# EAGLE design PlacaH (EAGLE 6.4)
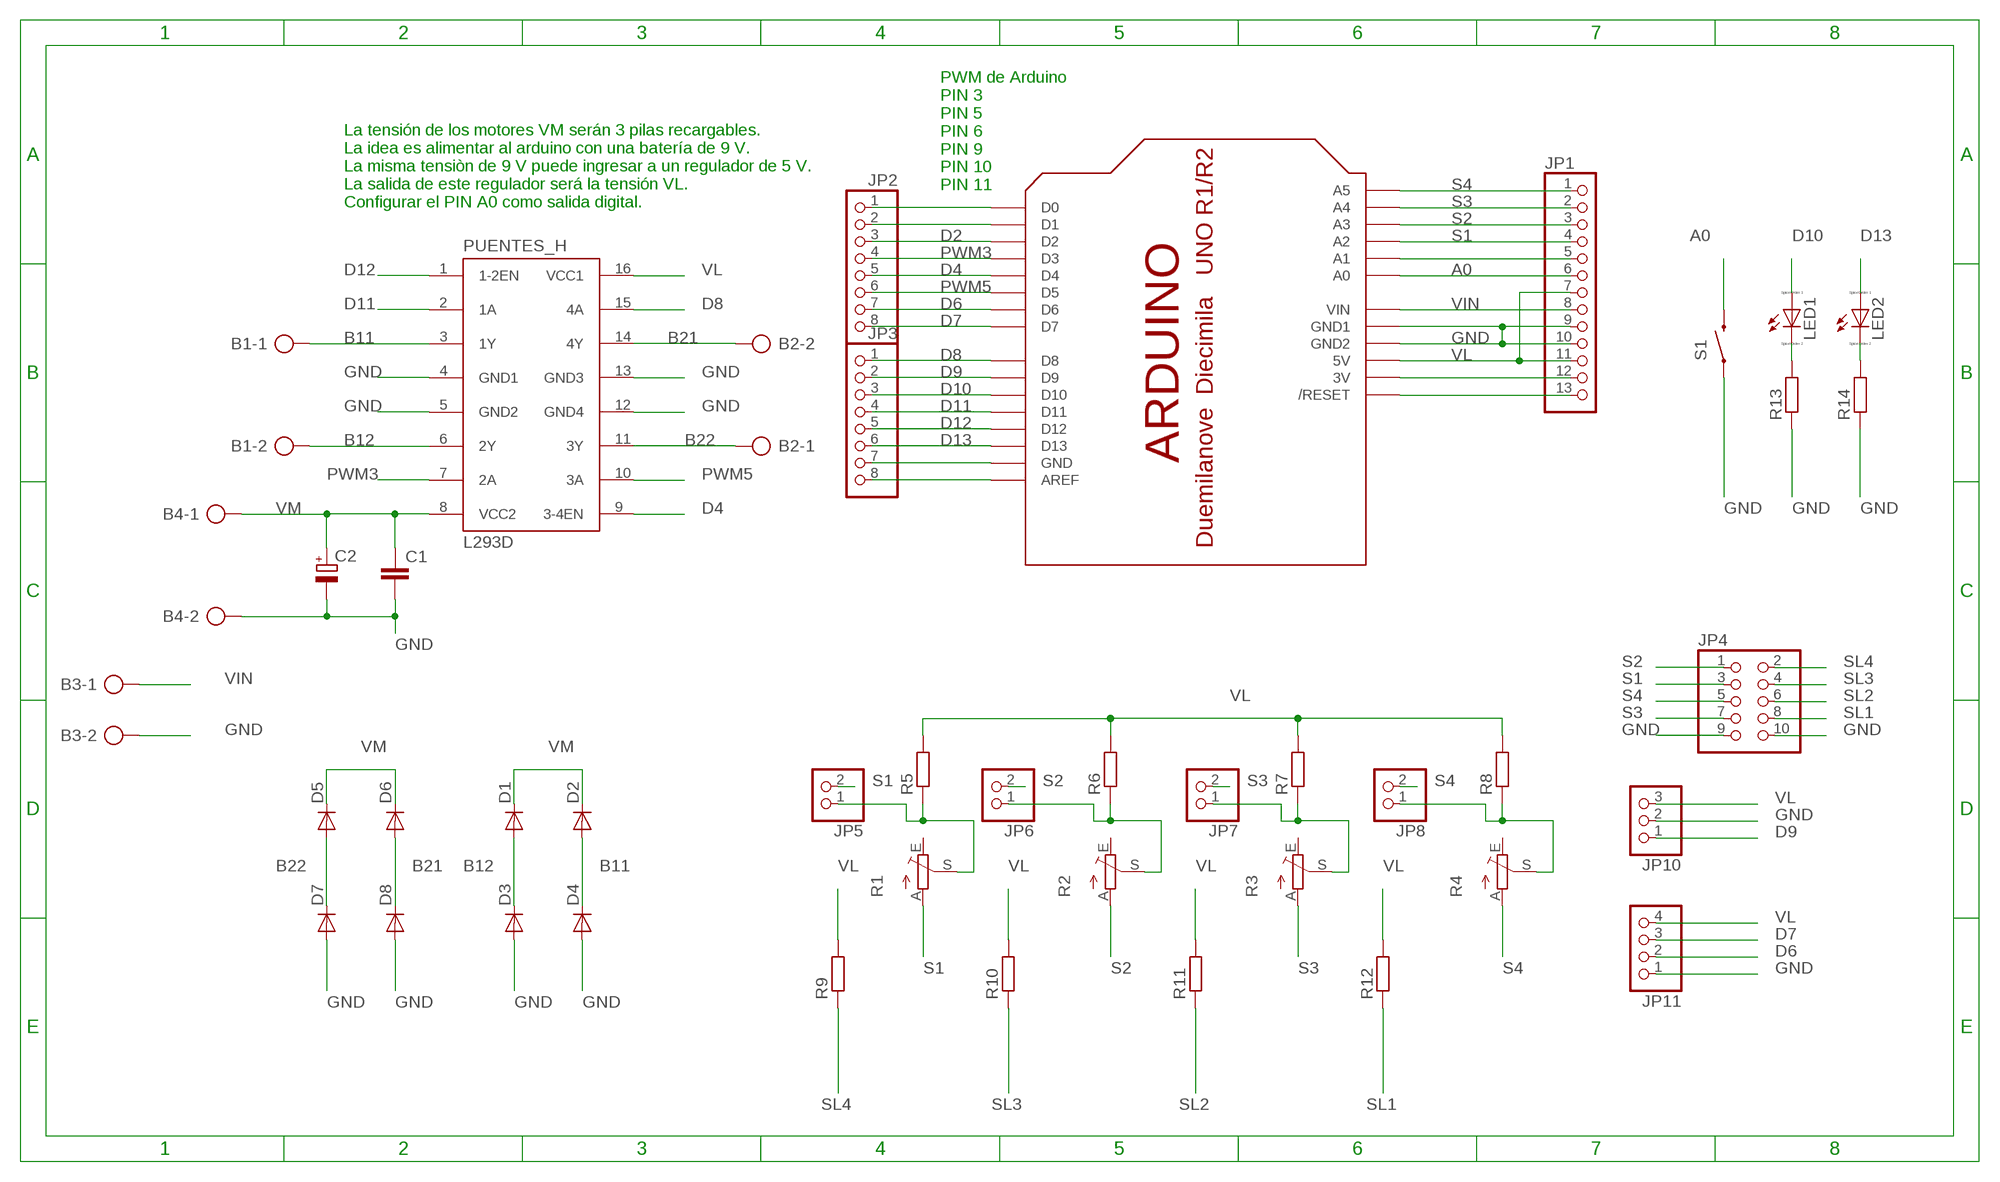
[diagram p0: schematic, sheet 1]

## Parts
B1  AK500/2-H  [AK500/2-H]
B2  AK500/2-H  [AK500/2-H]
B3  AK500/2-H  [AK500/2-H]
B4  AK500/2-H  [AK500/2-H]
C1  C-EUC1808  [C1808]
C2  CPOL-EUE2.5-6  [E2,5-6]
D1  CGRM4007-G  [SOD-123_MINI-SMA]
D2  CGRM4007-G  [SOD-123_MINI-SMA]
D3  CGRM4007-G  [SOD-123_MINI-SMA]
D4  CGRM4007-G  [SOD-123_MINI-SMA]
D5  CGRM4007-G  [SOD-123_MINI-SMA]
D6  CGRM4007-G  [SOD-123_MINI-SMA]
D7  CGRM4007-G  [SOD-123_MINI-SMA]
D8  CGRM4007-G  [SOD-123_MINI-SMA]
JP1  PINHD-1X13  [1X13]
JP2  PINHD-1X8  [1X08]
JP3  PINHD-1X8  [1X08]
JP4  PINHD-2X5  [2X05]
JP5  PINHD-1X2  [1X02]
JP6  PINHD-1X2  [1X02]
JP7  PINHD-1X2  [1X02]
JP8  PINHD-1X2  [1X02]
JP10  PINHD-1X3  [1X03]
JP11  PINHD-1X4  [1X04]
LED1  LED_E  [LED_1206]
LED2  LED_E  [LED_1206]
PUENTES_H  L293D  [DIL16]
R1  TRIM_EU-B25P  [B25P]
R2  TRIM_EU-B25P  [B25P]
R3  TRIM_EU-B25P  [B25P]
R4  TRIM_EU-B25P  [B25P]
R5  R-EU_M1206  [M1206]
R6  R-EU_M1206  [M1206]
R7  R-EU_M1206  [M1206]
R8  R-EU_M1206  [M1206]
R9  R-EU_M1206  [M1206]
R10  R-EU_M1206  [M1206]
R11  R-EU_M1206  [M1206]
R12  R-EU_M1206  [M1206]
R13  R-EU_M1206  [M1206]
R14  R-EU_M1206  [M1206]
S1  SWITCH-MOMENTARY-2PTH  [TACTILE-PTH]
U$1  ARDUINO-BPLACE  [ARDUINO-BPLACE]

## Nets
A0: JP1.6 S1.3 U$1.A0
B11: B1.1 D2.A D4.C PUENTES_H.3(1Y)
B12: B1.2 D1.A D3.C PUENTES_H.6(2Y)
B21: B2.2 D6.A D8.C PUENTES_H.14(4Y)
B22: B2.1 D5.A D7.C PUENTES_H.11(3Y)
D2: JP2.3 U$1.D2
D4: JP2.5 PUENTES_H.9(3-4EN) U$1.D4
D6: JP2.7 JP11.2 U$1.D6
D7: JP2.8 JP11.3 U$1.D7
D8: JP3.1 PUENTES_H.15(4A) U$1.D8
D9: JP3.2 JP10.1 U$1.D9
D10: JP3.3 LED1.A U$1.D10
D11: JP3.4 PUENTES_H.2(1A) U$1.D11
D12: JP3.5 PUENTES_H.1(1-2EN) U$1.D12
D13: JP3.6 LED2.A U$1.D13
GND: B3.2 B4.2 C1.2 C2.- D3.A D4.A D7.A D8.A JP1.9 JP1.10 JP4.9 JP4.10 JP10.2 JP11.1 PUENTES_H.4(GND1) PUENTES_H.5(GND2) PUENTES_H.12(GND4) PUENTES_H.13(GND3) R13.1 R14.1 S1.1 U$1.GND1 U$1.GND2
N$5: JP5.1 R1.S R5.1
N$7: JP6.1 R2.S R6.1
N$8: JP7.1 R3.S R7.1
N$9: JP8.1 R4.S R8.1
N$48: JP1.13 U$1.RESET(/RESET)
N$49: JP1.12 U$1.3V
N$51: JP1.5 U$1.A1
N$72: JP2.1 U$1.D0
N$73: JP2.2 U$1.D1
N$75: LED1.C R13.2
N$76: JP3.7 U$1.GND
N$77: JP3.8 U$1.AREF
N$163: LED2.C R14.2
PWM3: JP2.4 PUENTES_H.7(2A) U$1.D3
PWM5: JP2.6 PUENTES_H.10(3A) U$1.D5
S1: JP1.4 JP4.3 JP5.2 R1.A U$1.A2
S2: JP1.3 JP4.1 JP6.2 R2.A U$1.A3
S3: JP1.2 JP4.7 JP7.2 R3.A U$1.A4
S4: JP1.1 JP4.5 JP8.2 R4.A U$1.A5
SL1: JP4.8 R12.1
SL2: JP4.6 R11.1
SL3: JP4.4 R10.1
SL4: JP4.2 R9.1
VIN: B3.1 JP1.8 U$1.VIN
VL: JP1.7 JP1.11 JP10.3 JP11.4 PUENTES_H.16(VCC1) R5.2 R6.2 R7.2 R8.2 R9.2 R10.2 R11.2 R12.2 U$1.5V
VM: B4.1 C1.1 C2.+ D1.C D2.C D5.C D6.C PUENTES_H.8(VCC2)
Unconnected: R1.E R2.E R3.E R4.E

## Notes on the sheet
- PWM de Arduino
  PIN 3
  PIN 5
  PIN 6
  PIN 9
  PIN 10
  PIN 11
- La tensión de los motores VM serán 3 pilas recargables.
  La idea es alimentar al arduino con una batería de 9 V.
  La misma tensiòn de 9 V puede ingresar a un regulador de 5 V.
  La salida de este regulador será la tensión VL.
  Configurar el PIN A0 como salida digital.

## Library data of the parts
B1-B4 = con-ptr500:AK500/2-H: CONNECTOR; OC_FARNELL: unknown; OC_NEWARK: unknown
C1 = rcl:C-EU: CAPACITOR, European symbol
C2 = rcl:CPOL-EU: POLARIZED CAPACITOR, European symbol
D1-D8 = diode:CGRM400*-G: Molded plasitc,JEDEC SOD-123/Mini SMA
JP1 = pinhead:PINHD-1X13: PIN HEADER
JP2 JP3 = pinhead:PINHD-1X8: PIN HEADER
JP4 = pinhead:PINHD-2X5: PIN HEADER
JP5-JP8 = pinhead:PINHD-1X2: PIN HEADER
JP10 = pinhead:PINHD-1X3: PIN HEADER
JP11 = pinhead:PINHD-1X4: PIN HEADER
LED1 LED2 = eagle-ltspice:LED_E: LED; SPICEMODEL: NONE; SPICEPREFIX: D; SPICETYPE: diode
PUENTES_H = st-microelectronics:L293D: PUSH-PULL 4 CHANNEL DRIVER; MPN: L293D; OC_FARNELL: 9589619; OC_NEWARK: 56P8249
R1-R4 = pot:TRIM_EU-: POTENTIOMETER
R5-R14 = rcl:R-EU_: RESISTOR, European symbol
S1 = SparkFun-Electromechanical:SWITCH-MOMENTARY-2: Various NO switches- pushbuttons, reed, etc
U$1 = adafruit:ARDUINO: Arduino Diecimila/Duemilanove Make a shield with ease, this package has all the named pins as well as the two mounting drill holes and an outline of the USB and DC power connector. The outline is on the DIMENSION layer, so if your board house uses it they will cut the outline to match.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

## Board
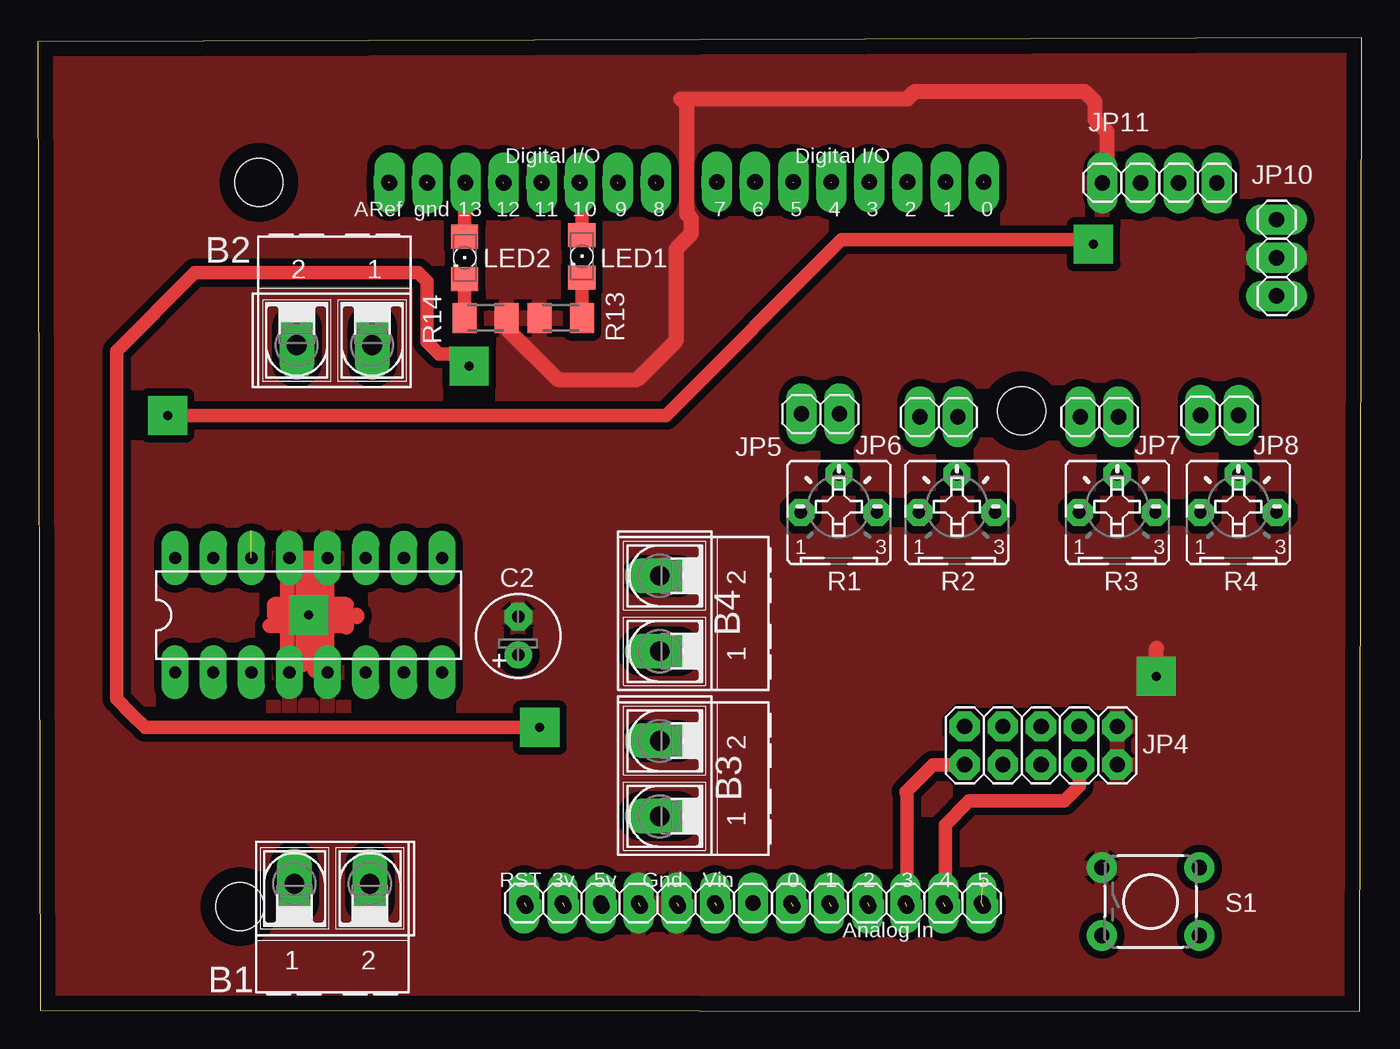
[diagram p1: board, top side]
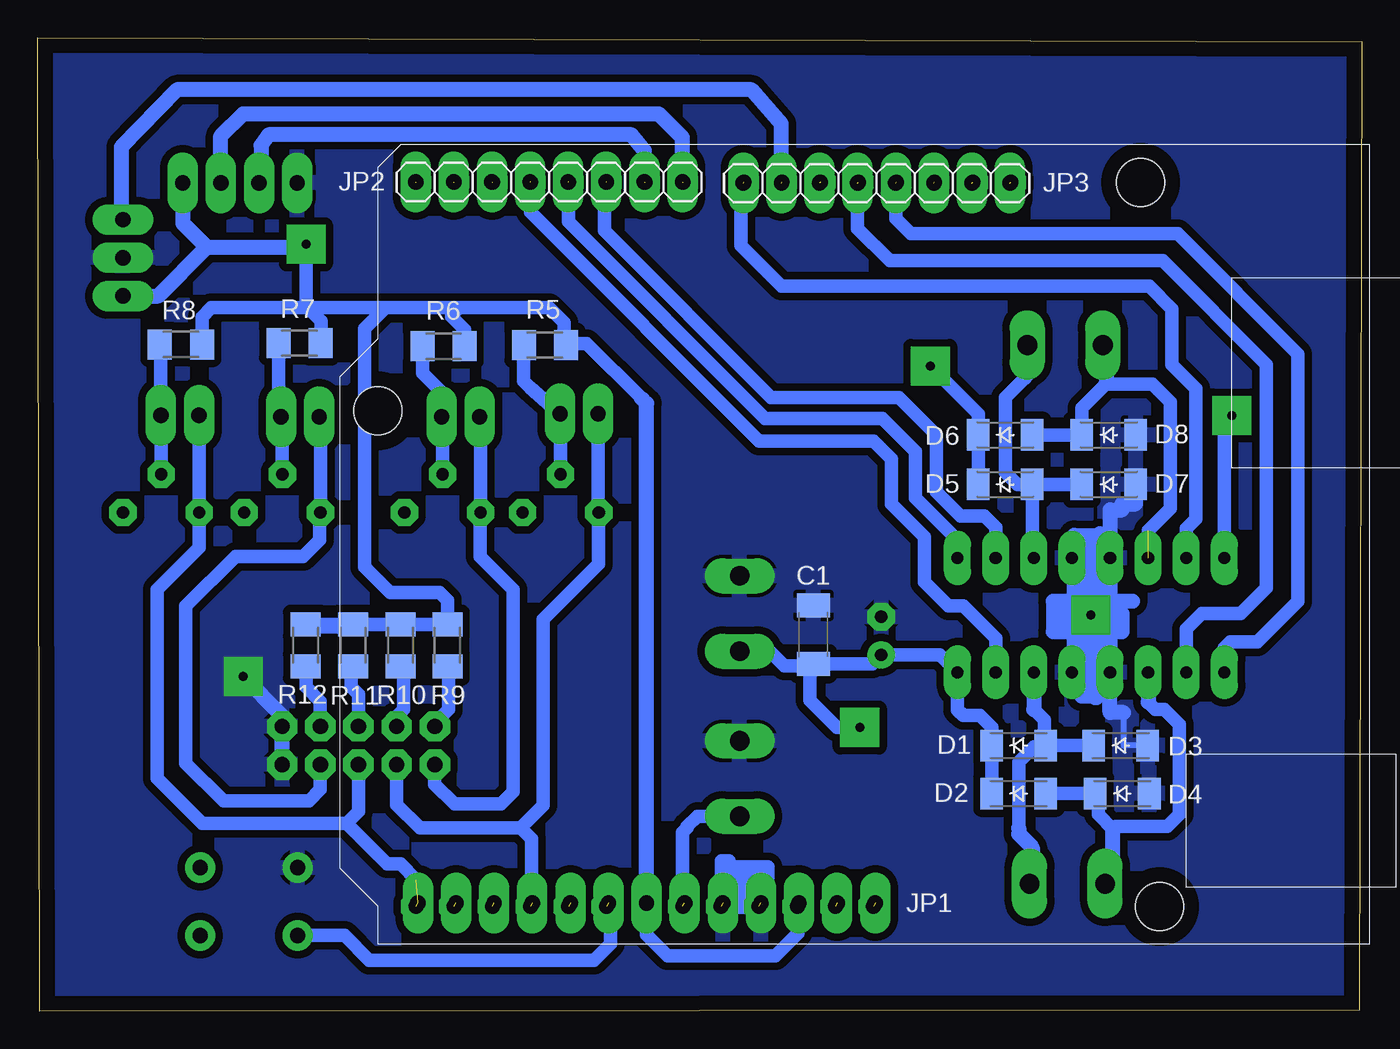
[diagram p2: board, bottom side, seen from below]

Size 88.26 x 64.91 mm. Coordinates in mm from the lower left corner, seen from the top.
Outline: 0.19,0.09 88.1,0 88.26,64.91 0,64.61 0.19,0.09
Copper layers (1*16): Top 0.035mm / dielectric 1.5mm / Bottom 0.035mm
Design rules "default *": minimum track width 1mm, minimum drill 0.01mm, track to track 0.5mm, track to pad 0.8mm, pad to pad 0.75mm, via to via 0.75mm, smd to smd 1mm, copper to edge 40mil, drill to drill 10mil, minimum pad ring 0.5mm, minimum via ring 1mm, stop-mask expansion 4mil, vias tented up to drill 0mil, thermal gap 10mil

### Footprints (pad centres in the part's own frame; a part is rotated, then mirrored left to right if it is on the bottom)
AK500/2-H = drill 1.321 long: 1 -2.515,0; 2 2.515,0
C1808 = smd 1.6 x 2.2: 1 -1.95,0; 2 1.95,0
E2,5-6 = drill 0.813 pad 1.6: + -1.27,0 | drill 0.813 pad 1.6 octagon: - 1.27,0
SOD-123_MINI-SMA = smd 1.5 x 2.1: A 1.8,0; C -1.8,0
1X13 = drill 1.016 long: 1 -15.24,0; 2 -12.7,0; 3 -10.16,0; 4 -7.62,0; 5 -5.08,0; 6 -2.54,0; 7 0,0; 8 2.54,0; 9 5.08,0; 10 7.62,0; 11 10.16,0; 12 12.7,0; 13 15.24,0
1X08 = drill 1.016 long: 1 -8.89,0; 2 -6.35,0; 3 -3.81,0; 4 -1.27,0; 5 1.27,0; 6 3.81,0; 7 6.35,0; 8 8.89,0
2X05 = drill 1.016 octagon: 1 -5.08,-1.27; 2 -5.08,1.27; 3 -2.54,-1.27; 4 -2.54,1.27; 5 0,-1.27; 6 0,1.27; 7 2.54,-1.27; 8 2.54,1.27; 9 5.08,-1.27; 10 5.08,1.27
1X02 = drill 1.016 long: 1 -1.27,0; 2 1.27,0
1X03 = drill 1.016 long: 1 -2.54,0; 2 0,0; 3 2.54,0
1X04 = drill 1.016 long: 1 -3.81,0; 2 -1.27,0; 3 1.27,0; 4 3.81,0
LED_1206 = smd 1.6 x 1.803: A -1.422,0; C 1.422,0
DIL16 = drill 0.813 long: 1 -8.89,-3.81; 2 -6.35,-3.81; 3 -3.81,-3.81; 4 -1.27,-3.81; 5 1.27,-3.81; 6 3.81,-3.81; 7 6.35,-3.81; 8 8.89,-3.81; 9 8.89,3.81; 10 6.35,3.81; 11 3.81,3.81; 12 1.27,3.81; 13 -1.27,3.81; 14 -3.81,3.81; 15 -6.35,3.81; 16 -8.89,3.81
B25P = drill 0.813 octagon: A -2.54,0; E 2.54,0; S 0,2.54
M1206 = smd 1.6 x 2: 1 -1.4,0; 2 1.4,0
TACTILE-PTH = drill 1.016 pad 1.88: 1 -3.251,2.261; 2 3.251,2.261; 3 -3.251,-2.261; 4 3.251,-2.261
ARDUINO-BPLACE = drill 1 pad 1.676 octagon: 3V 35.56,2.54; 5V 38.1,2.54; A0 50.8,2.54; A1 53.34,2.54; A2 55.88,2.54; A3 58.42,2.54; A4 60.96,2.54; A5 63.5,2.54; AREF 23.876,50.8; D0 63.5,50.8; D1 60.96,50.8; D2 58.42,50.8; D3 55.88,50.8; D4 53.34,50.8; D5 50.8,50.8; D6 48.26,50.8; D7 45.72,50.8; D8 41.656,50.8; D9 39.116,50.8; D10 36.576,50.8; D11 34.036,50.8; D12 31.496,50.8; D13 28.956,50.8; GND 26.416,50.8; GND1 43.18,2.54; GND2 40.64,2.54; RESET 33.02,2.54; VIN 45.72,2.54 | hole 3.2: 15.24,50.8; 66.04,35.56; 13.97,2.54

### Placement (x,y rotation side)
B1  19.63,8.51 0 top
B2  19.79,44.41 180 top
B3  41.47,15.52 90 top
B4  41.47,26.52 90 top
C1  36.56,25.11 90 bottom
C2  32.03,25.04 90 top
D1  22.87,17.72 0 bottom
D2  22.87,14.52 0 bottom
D3  16.07,17.72 0 bottom
D4  15.97,14.52 0 bottom
D5  23.77,35.12 0 bottom
D6  23.77,38.42 0 bottom
D7  16.87,35.12 0 bottom
D8  16.87,38.42 0 bottom
JP1  47.67,7.22 180 top
JP2  54.17,55.28 0 bottom
JP3  32.34,55.21 0 bottom
JP4  66.87,17.72 0 top
JP5  52.17,39.82 180 top
JP6  60.07,39.62 180 top
JP7  70.77,39.62 180 top
JP8  78.77,39.72 180 top
JP10  82.57,50.22 270 top
JP11  74.77,55.22 0 top
LED1  36.27,50.32 270 top
LED2  28.47,50.22 270 top
PUENTES_H  18.06,26.41 0 top
R1  53.4,33.26 0 top
R2  61.27,33.26 0 top
R3  71.95,33.26 0 top
R4  80.02,33.26 0 top
R5  54.45,44.4 0 bottom
R6  61.2,44.33 0 bottom
R7  70.8,44.55 0 bottom
R8  78.7,44.46 0 bottom
R9  60.95,24.41 90 bottom
R10  64.06,24.41 90 bottom
R11  67.23,24.41 90 bottom
R12  70.39,24.41 90 bottom
R13  34.87,46.22 0 top
R14  29.87,46.22 180 top
S1  74.17,7.32 0 top
U$1  -0.47,4.46 0 top

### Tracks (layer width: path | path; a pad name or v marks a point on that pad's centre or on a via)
A0  (1 unrouted)
  Bottom 0.9: S1.3 67.81,5.06 66.17,3.42 51.17,3.42 50.07,4.52 50.07,5.42 | 50.07,5.42 50.07,6.75 | JP1.6 50.21,5.56 50.07,5.42
B11
  Bottom 0.9: D2.A D4.C 17.57,14.32 17.57,13.12 16.59,12.14 16.41,12.32 12.97,12.32 12.17,13.12 12.17,19.12 13.17,20.12 13.77,20.12 14.25,20.6
  Bottom 1: PUENTES_H.3 14.25,20.6 | B1.1 16.59,8.51 16.59,12.14
B12
  Bottom 0.9: 21.87,20.12 21.17,19.42 21.17,17.82 D1.A | D1.A D3.C | 22.87,12.22 22.87,16.62 21.87,17.62 21.17,17.62 D1.A
  Bottom 1: PUENTES_H.6 21.87,20.12 | 21.62,8.51 B1.2 21.97,8.69 21.97,10.92 22.87,11.82 22.87,12.22
B21  (1 unrouted)
  Bottom 0.9: D6.A D8.C 18.67,40.22 17.04,41.86 17,41.82 13.97,41.82 12.77,40.62 12.77,33.52 14.25,32.04
  Bottom 1: B2.2 17.04,44.41 17.04,41.86
B22
  Bottom 0.9: D5.A 21.97,30.32 PUENTES_H.11 | D5.A D7.C | 22.07,42.63 22.47,42.22 23.77,40.92 23.77,35.92 22.97,35.12 D5.A
  Bottom 1: B2.1 22.47,44.41 22.47,42.22
D2  (1 unrouted)
D4  (1 unrouted)
  Bottom 0.9: PUENTES_H.9 26.95,31.4 29.77,34.22 29.77,37.32 31.97,39.52 39.77,39.52 52.87,52.62 U$1.D4
D6  (1 unrouted)
  Bottom 1: JP2.7 47.82,57.38 48.67,58.42 72.87,58.42 73.37,57.72 73.37,54.92 73.57,54.72 73.57,55.15 JP11.2
D7  (1 unrouted)
  Bottom 1: JP2.8 45.28,58.24 46.87,59.82 74.57,59.82 76.04,58.35 JP11.3
D8  (1 unrouted)
  Bottom 0.9: PUENTES_H.15 11.71,32.18 11.07,32.82 11.07,41.52 12.67,43.12 12.67,46.82 14.17,48.32 38.67,48.32 41.37,51.02 41.37,55.07 JP3.1
D9  (1 unrouted)
  Bottom 1: JP3.2 38.69,59.14 40.67,61.42 78.97,61.42 82.67,57.62 82.67,52.86 JP10.1
D10  (1 unrouted)
  Top 0.9: LED1.A 36.27,55.1 U$1.D10
D11  (1 unrouted)
  Bottom 0.9: PUENTES_H.2 11.71,25.48 10.67,26.52 8.07,26.52 6.37,28.22 6.37,43.12 13.27,50.02 31.47,50.02 33.61,52.16 JP3.4 33.57,55.17
D12  (1 unrouted)
  Bottom 0.9: PUENTES_H.1 9.17,24.22 8.77,24.62 6.97,24.62 4.27,27.32 4.27,43.82 12.27,51.82 30.07,51.82 31.07,52.82 JP3.5 | JP3.5
D13  (1 unrouted)
  Top 0.9: JP3.6 28.47,55.15 LED2.A
GND  (via drill 0.6)  (2 unrouted)
  Top 1: v74.57,22.32 74.57,24.22 | R14.1 31.27,45.52 34.67,42.12 39.97,42.12 42.57,44.72 42.57,50.82 43.57,51.82 43.57,52.82 43.27,53.12 43.27,60.42 42.87,60.82 57.97,60.82 58.47,61.32 69.77,61.32 70.47,60.62 70.47,59.42 71.27,58.62 71.27,55.53 JP11.1
  Bottom 0.406: PUENTES_H.4 PUENTES_H.5 | D3.A 15.87,17.72 15.87,19.92
  Bottom 0.9: PUENTES_H.5 19.17,22.6 19.17,26.62
  Bottom 1: PUENTES_H.12 16.77,30.22 | 15.87,19.92 16.79,19.92 PUENTES_H.4 PUENTES_H.13 16.67,30.22 16.77,30.22 | 16.77,30.22 16.77,33.42 15.97,33.42 15.97,33.82 15.07,33.82 D7.A | JP4.9 JP4.10 71.95,19.7 v74.57,22.32
  pour Bottom: 0.17,0.02 88.07,0.02 88.07,64.52 88.17,64.62 0.07,64.62 0.07,0.12
  pour Top: 0.17,0.02 88.07,0.02 88.07,64.82 0.07,64.82 0.07,0.12
N$2  (via drill 0.6)
  other vias: 18.07,26.42
N$3
  Bottom 1: 19.27,22.42 19.17,22.42 19.17,31.72 17.47,31.72 | 17.47,31.72 17.47,31.82 | 17.47,31.72 17.47,31.02 18.67,31.02 18.67,21.02 17.67,21.02 17.67,20.92 17.77,20.92 17.77,29.92
N$4
  Top 1: 20.57,27.12 15.77,27.12 15.77,26.42 21.27,26.42 21.27,26.32
N$5
  Bottom 0.9: R5.1 55.87,44.38 55.87,42.02 55.44,41.59 JP5.1 53.4,39.82 R1.S
N$7
  Bottom 0.9: R6.1 62.6,42.56 61.47,41.42 61.47,39.75 JP6.1 61.27,39.56 R2.S
N$8
  Bottom 0.9: R7.1 72.2,39.79 JP7.1 71.95,39.53 R3.S
N$9
  Bottom 0.9: R8.1 80.04,44.4 JP8.1 80.02,39.7 R4.S
N$16
  Top 1: 16.87,22.52 16.67,22.52 16.67,30.22 19.27,30.22 19.27,22.72 18.47,22.72 18.47,29.62 17.67,29.62 17.67,23.12
N$45
  Bottom 1: 15.27,27.32 20.57,27.32 20.57,25.32 15.97,25.32 15.97,26.52 19.97,26.52 19.97,25.92
N$46
  Bottom 1: 40.57,8.92 42.17,8.92 42.17,8.42 40.37,8.42
N$48  (1 unrouted)
N$49  (1 unrouted)
N$50
  Top 1: 20.57,25.62 20.57,25.72 15.47,25.72
N$51  (1 unrouted)
N$52
  Bottom 0.9: 42.57,7.02 42.67,7.02 42.67,10.02 42.17,10.02 42.17,9.62 39.57,9.62 39.57,8.92 40.07,8.92 40.07,6.92 42.57,6.92 42.57,7.52 40.77,7.52 40.77,7.62
N$72  (1 unrouted)
N$73  (1 unrouted)
N$75
  Top 0.9: LED1.C R13.2
N$76  (1 unrouted)
N$77  (1 unrouted)
N$163
  Top 0.9: LED2.C R14.2
PWM3  (1 unrouted)
  Bottom 0.9: PUENTES_H.7 24.41,24.86 26.57,27.02 27.57,27.02 29.17,28.62 29.17,31.62 31.37,33.82 31.37,36.82 32.57,38.02 40.17,38.02 55.41,53.26 U$1.D3
PWM5  (1 unrouted)
  Bottom 0.9: PUENTES_H.10 24.41,32.26 25.17,33.02 26.77,33.02 28.37,34.62 28.37,38.42 30.87,40.92 39.37,40.92 50.47,52.02 50.47,55.12 U$1.D5
S1  (1 unrouted)
  Bottom 0.9: JP4.3 64.33,13.78 62.77,12.22 56.07,12.22 | 56.07,12.22 54.57,13.72 54.57,26.12 50.87,29.82 R1.A 50.9,33.26 JP5.2 | 56.07,12.22 55.34,11.49 55.34,7.27 JP1.4
S2  (1 unrouted)
  Top 0.9: JP4.1 61.76,16.42 59.67,16.42 57.88,14.63 57.95,14.56 U$1.A3
  Bottom 0.9: JP4.1 61.79,15.14 60.47,13.82 57.37,13.82 56.57,14.62 56.57,28.12 58.77,30.32 58.77,33.22 R2.A 58.73,39.56 JP6.2
S3  (1 unrouted)
  Top 0.9: JP4.7 69.41,15.02 68.41,14.02 62.07,14.02 60.49,12.44 U$1.A4
  Bottom 0.9: JP4.7 69.41,14.78 70.17,14.02 75.87,14.02 78.37,16.52 78.37,27.02 75.07,30.32 70.57,30.32 69.47,31.42 69.47,33.19 R3.A 69.41,39.79 69.07,40.12 69.07,40.05 JP7.2
S4  (2 unrouted)
  Bottom 0.9: JP4.5 66.87,13.32 67.67,12.52 | 67.67,12.52 77.27,12.52 80.27,15.52 80.27,28.12 77.47,30.92 R4.A 77.48,39.7 JP8.2 | 63.03,8.78 64.07,9.82 64.97,9.82 67.67,12.52
SL1
  Bottom 0.9: JP4.8 69.41,20.66 70.37,21.62 70.37,22.98 R12.1
SL2
  Bottom 0.9: JP4.6 66.87,21.12 67.37,21.62 67.37,22.86 R11.1
SL3
  Bottom 0.9: JP4.4 64.33,19.66 63.87,20.12 63.87,22.81 R10.1
SL4
  Bottom 0.9: JP4.2 61.79,19.2 60.87,20.12 60.87,22.93 R9.1
VIN  (1 unrouted)
  Bottom 0.9: B3.1 44.29,13.01 44.97,12.32 44.97,12.22 45.27,11.92 45.27,7.72 | 45.27,7.72 45.27,7.03 | U$1.VIN 45.25,7.7 45.27,7.72
VL  (via drill 0.6)
  Top 0.9: v8.67,39.72 41.87,39.72 53.57,51.42 70.07,51.42 v70.37,51.12
  Bottom 0.9: R11.2 R12.2 70.39,25.65 70.37,25.62 67.41,25.62 R11.2 | R11.2 R10.2 R9.2 60.95,27.4 61.47,27.92 64.77,27.92 66.47,29.62 66.47,45.52 65.07,46.92 | 70.67,46.92 76.67,46.92 77.3,46.29 R8.2 | 70.67,46.92 70.27,46.92 | 70.27,46.92 69.37,46.02 69.37,44.58 R7.2 | 70.27,46.92 65.07,46.92 | 65.07,46.92 60.17,46.92 | 60.17,46.92 54.17,46.92 53.17,45.92 53.17,44.52 R5.2 52.93,44.52 51.67,44.52 48.02,40.87 47.72,40.57 | 60.17,46.92 60.67,46.42 60.67,46.32 59.8,45.46 R6.2 | PUENTES_H.16 9.17,39.22 v8.67,39.72 | v70.37,51.12 70.37,47.22 70.67,46.92 | JP1.7 47.67,5.12 46.27,3.72 39.07,3.72 37.57,5.22 37.57,5.62 | 37.57,5.62 37.57,6.95 U$1.5V | JP1.11 37.51,5.68 37.57,5.62
  Bottom 1: JP11.4 78.58,52.53 76.97,50.92 | 76.97,50.92 70.57,50.92 v70.37,51.12 | JP10.3 80.21,47.68 76.97,50.92 | JP1.7 47.67,40.52 48.02,40.87
VM  (via drill 0.6)
  Top 0.9: v28.77,43.02 28.77,43.32 28.27,43.82 26.77,43.82 25.97,44.62 25.97,48.62 25.37,49.22 10.47,49.22 5.27,44.02 5.27,20.82 6.22,19.87 7.17,18.92 v33.47,18.92
  Bottom 0.9: D2.C D1.C 24.67,18.92 25.47,19.72 26.57,19.72 26.95,20.1 PUENTES_H.8 28.11,23.77 C2.+ 32.64,23.16 36.07,23.16 | B4.1 39.46,24.01 38.47,23.02 36.7,23.02 C1.1 36.07,23.16 | D6.C D5.C 25.57,39.82 v28.77,43.02 | v33.47,18.92 34.97,18.92 36.77,20.72 36.77,22.46 36.07,23.16

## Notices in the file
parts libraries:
SparkFun-Electromechanical: Licensing: CC v3.0 Share-Alike You are welcome to use this library for commercial purposes.
